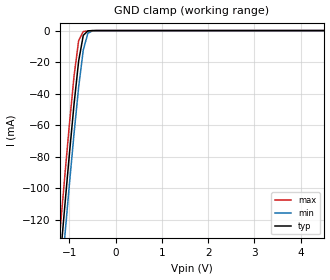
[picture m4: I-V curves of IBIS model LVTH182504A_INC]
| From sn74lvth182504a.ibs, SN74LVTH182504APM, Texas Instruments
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[Model]   LVTH182504A_INC
| high-impedance input buffer
| iclk.lvta (97212 ALEY)
| pad.lvta  (97212 ALEY)
| Signals   CLK, CLKEN#, LE
Model_type  Input
Polarity   Non-Inverting
Vinl = 0.8V
Vinh = 2.0V
| variable   typ   min   max
C_comp   4p   NA   NA
[Temperature Range]   50   100   0
[Voltage range]   3.3   3   3.6
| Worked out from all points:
|   GND clamp passes 1 mA (typ) near -0.63 V on its own axis
|Process range|   weak   strong
[gnd_clamp]
|   50C:3.3V:   100C:3V:weak   0C:3.6V:strong
|   Voltage   I(typ)   I(min)   I(max)
-3.3V     -902.8mA   -920.5mA   -885.5mA
-1.2V     -145.7mA   -165.1mA   -126.6mA
-1.1V     -111.6mA   -131mA     -92.49mA
-1V       -78.36mA   -97.58mA   -59.49mA
-900mV    -46.84mA   -65.49mA   -29.02mA
-800mV    -19.33mA   -35.9mA    -6.331mA
-700mV    -3.025mA   -12.3mA    -602.9uA
-600mV    -177.8uA   -1.693mA   -229.1uA
-500mV    -5.2uA     -126.4uA   -50.31uA
6.6V      1.98nA     2.082nA    1.98nA
